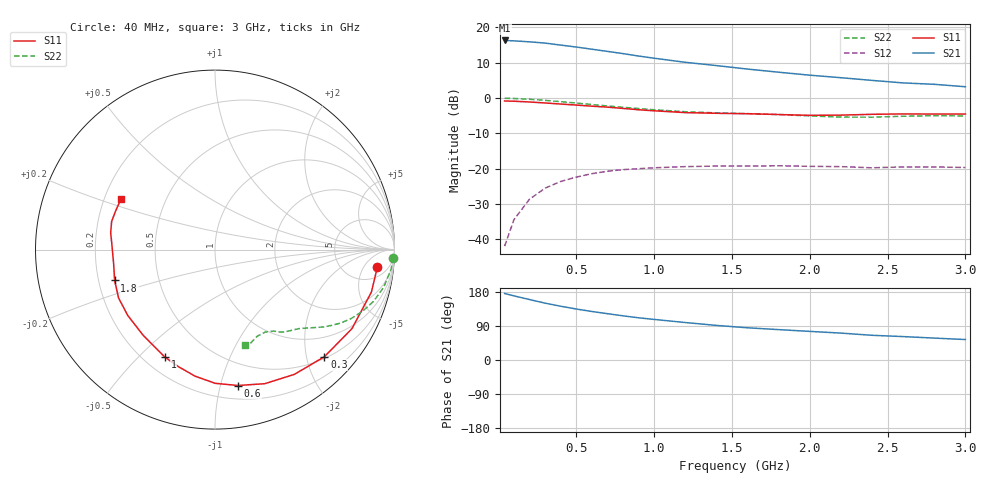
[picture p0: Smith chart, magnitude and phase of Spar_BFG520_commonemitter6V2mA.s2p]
! Filename:  BFG520G.S2P  Version:  2.1
! NXP part #: BFG520  Date: Feb 1992
! Bias condition: Vce=6V, Ic=2mA
! IN LINE PINNING: same data as with cross emitter pinning.
#  MHz  S  MA  R  50
! Freq  S11  S21  S12  S22  !GUM [dB]
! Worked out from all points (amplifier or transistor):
!   21 points, 40 MHz to 3 GHz, reference 50 ohm
!   highest |S21| = 16.3 dB at 40 MHz (marker M1)
!   |S21| within 3 dB of that: start of sweep to 685.6 MHz
!   unconditionally stable (mu >= 1): 2.296 GHz to end of sweep
!   at 300 MHz: K = 0.10, MSG = 20.5 dB, |S12| = -25.5 dB
!   at 1 GHz: K = 0.37, MSG = 15.5 dB, |S12| = -19.7 dB
!   at 3 GHz: K = 1.23, MAG = 8.6 dB, |S12| = -19.7 dB
!   S11 on the Smith chart (normalised r, x): 40 MHz: 9, -11; 300 MHz: 0.54, -2.35; 600 MHz: 0.31, -1.14; 1 GHz: 0.28, -0.60; 1.8 GHz: 0.27, -0.14; 3 GHz: 0.27, +0.23
40  0.91 -6.1  6.548 175.5  0.008 84.5  0.994 -2.6
100  0.903 -15.2  6.463 169.3  0.019 81.8  0.987 -6.5
200  0.881 -30.0  6.26 159.5  0.037 73.5  0.963 -12.6
300  0.853 -44.4  6.009 150.0  0.053 66.4  0.929 -18.1
400  0.824 -57.5  5.629 141.9  0.066 60.2  0.89 -22.8
500  0.797 -69.6  5.286 134.6  0.076 54.4  0.85 -26.9
600  0.768 -80.4  4.922 128.0  0.085 49.7  0.811 -30.3
700  0.745 -89.9  4.589 122.3  0.092 45.7  0.774 -33.1
800  0.714 -98.9  4.268 116.6  0.097 42.3  0.742 -35.5
900  0.684 -107.1  3.941 111.4  0.1 39.5  0.711 -37.6
1000  0.661 -115.0  3.672 107.1  0.103 37.2  0.684 -39.6
1200  0.623 -130.0  3.213 98.9  0.107 33.3  0.641 -43.4
1400  0.609 -143.0  2.888 91.3  0.109 30.1  0.617 -47.0
1600  0.601 -153.4  2.576 85.0  0.109 29.7  0.602 -49.6
1800  0.585 -162.9  2.326 80.2  0.11 29.2  0.585 -51.7
2000  0.57 -172.4  2.111 75.5  0.108 28.8  0.559 -54.3
2200  0.574 178.1  1.944 71.0  0.107 28.8  0.538 -58.7
2400  0.589 170.7  1.781 65.2  0.103 29.7  0.537 -64.0
2600  0.597 164.7  1.64 61.8  0.106 31.9  0.553 -68.2
2800  0.594 158.8  1.567 57.8  0.106 33.1  0.564 -70.4
3000  0.595 151.9  1.448 54.0  0.104 36.6  0.558 -72.4
